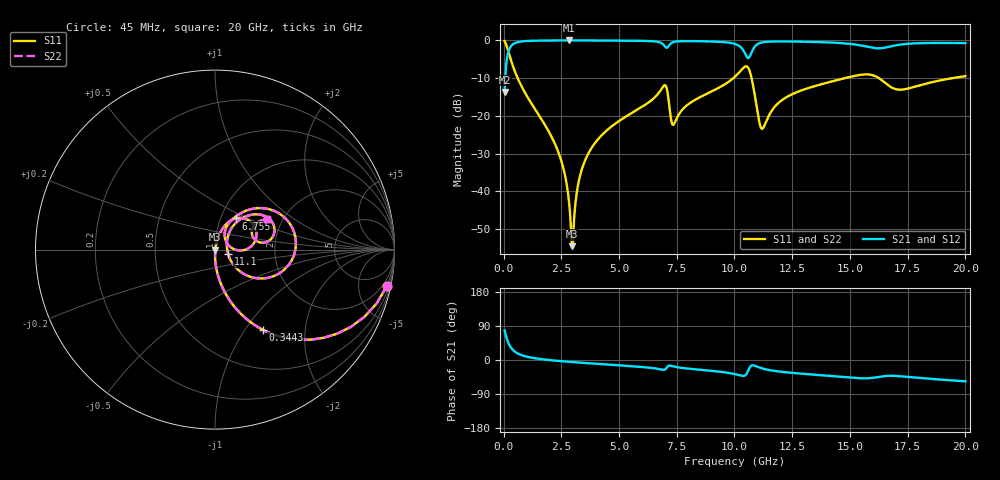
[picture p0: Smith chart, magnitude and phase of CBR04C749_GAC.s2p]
! S-parameter model data by Modelithics Inc.  support@modelithics.com 813-866-6335  Tampa FL USA
! S-Parameter data specifications:
! Substrate: 20-mil Rogers 4350B, substrate thickness, H=0.508mm, Dielectric constant, Er=3.75
! PCB Mounting Pad Footprint: Pad width, PadW=0.52mm , Pad length, PadL=0.52mm , Pad gap, PadG (edge-to-edge)=0.28mm , Reference planes=1.32mm apart
#  GHz  S  MA  R 50
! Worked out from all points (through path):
!   801 points, 45 MHz to 20 GHz, reference 50 ohm
!   highest |S21| = -0.02 dB at 2.814 GHz (marker M1); lowest = -13.7 dB at 45 MHz (marker M2)
!   group delay of S21, straight-line fit = 9.14 ps
!   lowest |S11| = -54.6 dB at 2.963 GHz (marker M3), VSWR 1.00, Z = 50.2 - j0.0666 ohm
!   |S11| at or under -10 dB: 609.9 MHz to 9.952 GHz (9.342 GHz wide, 177 % of centre); 10.74 GHz to 14.78 GHz (4.045 GHz wide, 31.7 % of centre); 16.25 GHz to 19.45 GHz (3.194 GHz wide, 17.9 % of centre)
!   |S22| runs from -54.6 to -0.2 dB; largest |S21 - S12| = 0
!   S11 on the Smith chart (normalised r, x): 45 MHz: 0.99, -9.36; 344.3 MHz: 0.99, -1.21; 6.755 GHz: 1.18, +0.43; 11.1 GHz: 1.16, -0.06; 20 GHz: 1.67, +0.64
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0.045  0.9782 -12.1  0.2075 77.9  0.2075 77.9  0.9782 -12.1
0.194662  0.7353 -43.0  0.6774 47.0  0.6774 47.0  0.7353 -43.0
0.344325  0.5193 -59.3  0.854 30.7  0.854 30.7  0.5193 -59.3
0.8432  0.2257 -78.3  0.9732 11.5  0.9732 11.5  0.2257 -78.3
2.289938  0.03823 -89.6  0.9976 -2.0  0.9976 -2.0  0.03823 -89.6
2.614206  0.01885 -88.6  0.9981 -3.7  0.9981 -3.7  0.01885 -88.6
2.813756  0.008249 -82.4  0.9981 -4.7  0.9981 -4.7  0.008249 -82.4
2.963419  0.001871 -20.8  0.9981 -5.4  0.9981 -5.4  0.001871 -20.8
3.387462  0.01941 76.9  0.9978 -7.3  0.9978 -7.3  0.01941 76.9
4.285437  0.05674 76.6  0.9959 -11.1  0.9959 -11.1  0.05674 76.6
6.704981  0.1986 58.7  0.9536 -23.6  0.9536 -23.6  0.1986 58.7
6.754869  0.208 56.5  0.9448 -24.2  0.9448 -24.2  0.208 56.5
7.02925  0.2488 21.6  0.807 -22.9  0.807 -22.9  0.2488 21.6
7.378463  0.07769 39.5  0.9549 -17.2  0.9549 -17.2  0.07769 39.5
10.0225  0.3306 44.3  0.897 -37.4  0.897 -37.4  0.3306 44.3
10.34677  0.4208 26.5  0.7654 -41.9  0.7654 -41.9  0.4208 26.5
10.59621  0.4322 -7.7  0.5828 -27.9  0.5828 -27.9  0.4322 -7.7
11.09508  0.07785 -19.3  0.9218 -20.3  0.9218 -20.3  0.07785 -19.3
13.36496  0.242 48.2  0.9553 -38.4  0.9553 -38.4  0.242 48.2
15.68473  0.3542 23.8  0.8322 -48.3  0.8322 -48.3  0.3542 23.8
16.68248  0.2509 9.3  0.8225 -41.7  0.8225 -41.7  0.2509 9.3
20  0.3362 30.2  0.9203 -56.2  0.9203 -56.2  0.3362 30.2
